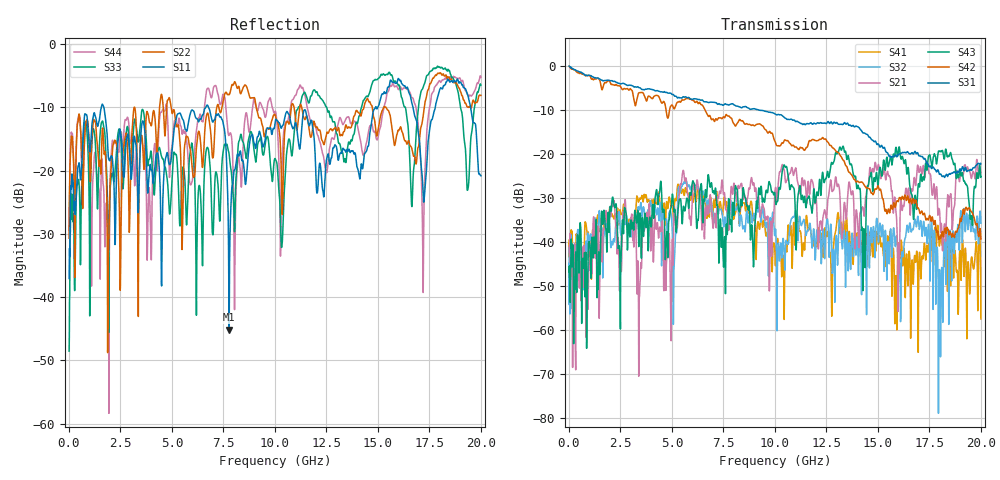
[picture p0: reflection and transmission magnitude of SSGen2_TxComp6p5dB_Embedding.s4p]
! C:\Users\lab_ccd01\Downloads\USBIF_6p5dB_at_5GHz_new_1.s4p
! Sun Feb 23 15:10:50 2025
!!Measured using Teledyne LeCroy WavePulser LCRY4802N20219
!MixedMode
!DutToConverterPinDefinitions,+1,-1,+2,-2
!UserPortDefinitions,D1,C1,D2,C2
! freq S11 S12 S13 S14
! S21 S22 S23 S24
! S31 S32 S33 S34
! S41 S42 S43 S44
# GHz S MA R 50.00
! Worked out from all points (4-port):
!   2000 points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, 10 MHz to 20 GHz, reference 50 ohm
!   strongest paths, dB at 10 MHz, 5.01 GHz, 10.01 GHz, 15.01 GHz, 20 GHz:
!     S31: -0.1, -6.6, -11.0, -17.8, -22.3
!     S42: -0.2, -9.0, -17.3, -27.3, -39.4
!     S43: -46.9, -29.4, -29.5, -27.2, -25.2
!     S21: -40.8, -40.7, -28.3, -22.6, -24.4
!     S32: -41.3, -36.6, -37.7, -38.9, -35.8
!     S41: -39.6, -31.9, -43.7, -39.9, -57.5
!   lowest |S11| = -45.2 dB at 7.78 GHz (marker M1), VSWR 1.01, Z = 49.6 - j0.379 ohm
!   |S11| at or under -10 dB: start of sweep to 1.572 GHz; 1.696 GHz to 6.641 GHz (4.945 GHz wide, 119 % of centre); 6.774 GHz to 14.88 GHz (8.106 GHz wide, 74.9 % of centre)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
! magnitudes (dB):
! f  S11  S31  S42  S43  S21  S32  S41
! 10 MHz  -37.1  -0.1  -0.2  -46.9  -40.8  -41.3  -39.6
! 790 MHz  -11.0  -2.2  -2.3  -52.5  -43.4  -45.5  -35.5
! 7.31 GHz  -11.5  -8.7  -11.9  -38.6  -28.5  -32.6  -31.6
! 7.78 GHz  -45.2  -9.0  -11.5  -31.3  -36.1  -32.6  -31.3
! 16.38 GHz  -7.0  -19.8  -30.6  -23.4  -27.9  -37.6  -43.2
! 17.19 GHz  -23.1  -20.9  -33.9  -25.3  -22.9  -36.4  -43.9
! 20 GHz  -20.8  -22.3  -39.4  -25.2  -24.4  -35.8  -57.5
